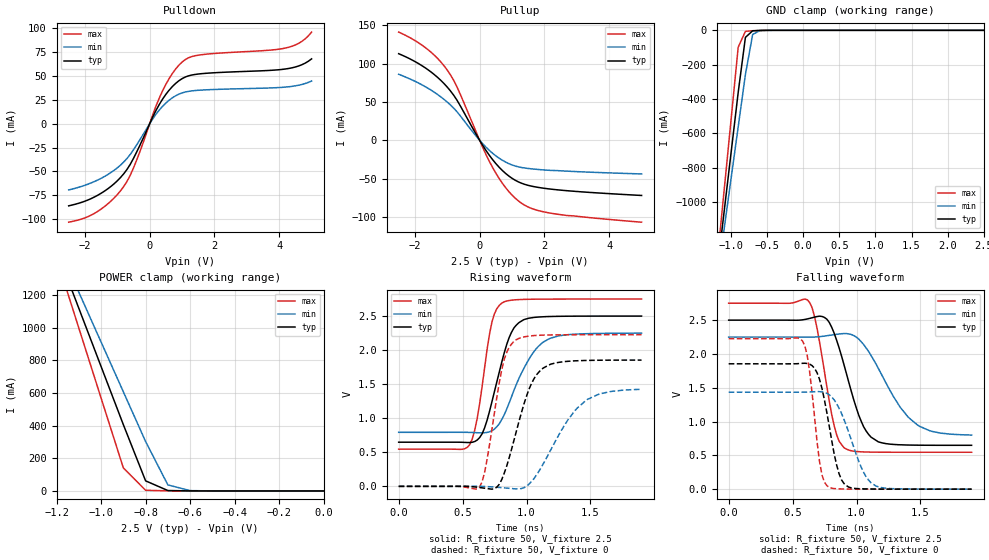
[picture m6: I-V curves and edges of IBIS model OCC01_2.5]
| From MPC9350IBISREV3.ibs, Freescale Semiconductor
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|   OCC01_2.5: LVCMOS OUTPUT MODEL
[Model]   OCC01_2.5
Model_type  3-state
Enable   Active-Low
Polarity   Non-Inverting
Vmeas   =   1.25
C_comp   3.5pF   3.5pF   3.5pF
[Temperature Range] 55   110   0
[Voltage Range]   2.5   2.25   2.75
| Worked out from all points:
|   slope of the pulldown table from 0 to 0.375 V, typ, clamps not added: 15.3 ohm
|   slope of the pullup table from 0 to 0.375 V, typ, clamps not added: 15.8 ohm
|   GND clamp passes 1 mA (typ) near -0.62 V on its own axis
|   POWER clamp passes 1 mA (typ) near -0.64 V on its own axis
|   falling waveform, R_fixture 50, V_fixture 2.5: 20-80 % time 177ps typ, 274ps min, 122ps max; typ from 2.5 V to 0.649 V
|   falling waveform, R_fixture 50, V_fixture 0: 20-80 % time 112ps typ, 170ps min, 78.4ps max; typ from 1.85 V to 0 V
|   rising waveform, R_fixture 50, V_fixture 2.5: 20-80 % time 155ps typ, 217ps min, 105ps max; typ from 0.649 V to 2.5 V
|   rising waveform, R_fixture 50, V_fixture 0: 20-80 % time 176ps typ, 276ps min, 119ps max; typ from 0 V to 1.85 V
[Pullup]
-2.5V     113.1mA    86.24mA    141.3mA
-1.6V     92.3mA     68.09mA    118.5mA
-1.3V     82.22mA    59.86mA    107mA
-1V       69.48mA    49.91mA    91.73mA
-700mV    52.4mA     37.33mA    69.8mA
0V        0A         1fA        0A
400mV     -25.19mA   -16.89mA   -35.45mA
800mV     -43.17mA   -28.34mA   -61.65mA
1.2V      -54.33mA   -34.65mA   -79.21mA
1.6V      -59.78mA   -37.22mA   -88.87mA
2.2V      -63.7mA    -39.27mA   -95.12mA
5V        -71.96mA   -43.87mA   -106.9mA
[Pulldown]
-2.5V     -85.99mA   -69.34mA   -103.1mA
-1.6V     -74.82mA   -58.88mA   -91.7mA
-1.2V     -65.76mA   -51.2mA    -81.14mA
-800mV    -52.4mA    -40.08mA   -65.69mA
-500mV    -36.35mA   -27.29mA   -46.41mA
400mV     25.85mA    18.3mA     34.56mA
700mV     38.92mA    27.15mA    52.55mA
1V        47.23mA    32.3mA     64.6mA
1.6V      52.46mA    35.28mA    72.32mA
4.2V      57.42mA    38.45mA    79.38mA
4.7V      61.86mA    41.16mA    86.31mA
5V        68mA       44.83mA    96.03mA
[GND Clamp]
-2.5V     -6.069A    -5.45A     -6.952A
-1.2V     -1.43A     -1.477A    -1.382A
-1.1V     -1.074A    -1.171A    -953.9mA
-1V       -717.3mA   -866.4mA   -525.7mA
-900mV    -361.1mA   -561.5mA   -98.15mA
-800mV    -41.01mA   -256.9mA   -6.004mA
-700mV    -2.888mA   -24.01mA   -2.342mA
-600mV    -641.5uA   -1.609mA   -734.7uA
2.5V      190.6pA    157.5nA    24.14pA
[POWER Clamp]
-2.5V     6.133A     5.506A     7.023A
-1.2V     1.476A     1.523A     1.427A
-1.1V     1.119A     1.217A     998mA
-1V       762.3mA    912.1mA    569.3mA
-900mV    406mA      607.2mA    141.1mA
-800mV    61.63mA    302.7mA    3.873mA
-700mV    2.356mA    36.76mA    461.2uA
-600mV    158.8uA    1.918mA    48.48uA
0V        190.6pA    891.7pA    28.09pA
[Falling Waveform]
R_fixture=50
V_fixture=2.5
V_fixture_min=2.25
V_fixture_max=2.75
0s        2.5V       2.25V      2.75V
633.3ps   2.526V     2.248V     2.761V
690.9ps   2.553V     2.252V     2.382V
786.9ps   2.466V     2.275V     1.301V
844.4ps   2.202V     2.29V      804mV
902ps     1.84V      2.301V     613.2mV
1.056ns   923.1mV    2.139V     550.7mV
1.171ns   699.6mV    1.786V     546.9mV
1.478ns   650.7mV    948mV      545.8mV
1.9ns     648.5mV    800.2mV    545.8mV
[Falling Waveform]
R_fixture=50
V_fixture=0
V_fixture_min=0
V_fixture_max=0
0s        1.854V     1.434V     2.226V
575.8ps   1.861V     1.435V     2.196V
633.3ps   1.849V     1.438V     1.733V
690.9ps   1.723V     1.443V     710.4mV
729.3ps   1.494V     1.439V     212.4mV
786.9ps   928.3mV    1.396V     25.8mV
882.8ps   136.8mV    1.12V      3.229mV
1.036ns   5.326mV    324.2mV    406.1uV
1.113ns   2.358mV    93.83mV    150uV
1.9ns     1.401uV    112.2uV    37.77nV
[Rising Waveform]
R_fixture=50
V_fixture=2.5
V_fixture_min=2.25
V_fixture_max=2.75
0s        648.5mV    793.4mV    545.8mV
556.6ps   643.8mV    792.2mV    614.9mV
614.1ps   679.9mV    787.7mV    997.8mV
671.7ps   857mV      787.2mV    1.735V
729.3ps   1.242V     817.5mV    2.412V
806.1ps   1.823V     981.4mV    2.691V
863.6ps   2.183V     1.222V     2.728V
921.2ps   2.37V      1.501V     2.74V
1.132ns   2.49V      2.12V      2.749V
1.9ns     2.5V       2.249V     2.75V
[Rising Waveform]
R_fixture=50
V_fixture=0
V_fixture_min=0
V_fixture_max=0
0s        1.374nV    11.02nV    122.5pV
633.3ps   -17.33mV   534.6uV    -8.548mV
690.9ps   -32.07mV   -3.315mV   389.2mV
767.7ps   -12.34mV   -13.06mV   1.309V
825.3ps   192.3mV    -22.44mV   1.863V
921.2ps   814.1mV    -37.94mV   2.154V
1.017ns   1.417V     27.39mV    2.206V
1.132ns   1.739V     336.3mV    2.221V
1.459ns   1.848V     1.251V     2.226V
1.9ns     1.854V     1.425V     2.226V
[Ramp]
R_load=50
dV/dt_r   1.112E+0/1.757E-10   8.551E-1/2.740E-10   1.336E+0/1.182E-10
dV/dt_f   1.111E+0/1.757E-10   8.699E-1/2.744E-10   1.323E+0/1.212E-10
|[End   OCC01_2.5
